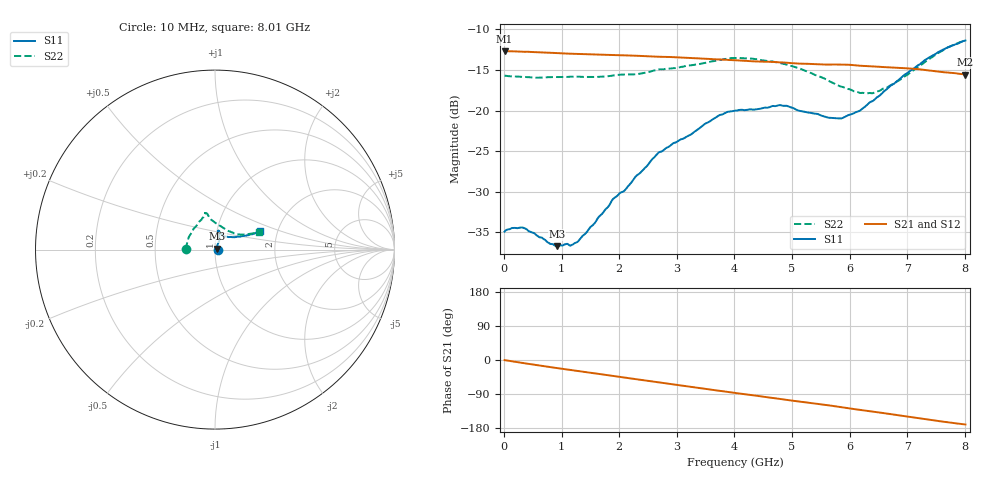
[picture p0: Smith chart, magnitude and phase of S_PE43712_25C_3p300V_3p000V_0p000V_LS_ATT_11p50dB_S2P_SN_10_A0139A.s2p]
! DEVICE ID: PE43712
! File Path: z:\PE43713\PE43713_CHAR_NOM_04292014\AMB\3p300\LS_ATT_11p50dB\PE43713_AMB_3p300V_3p000V_0p000V_LS_ATT_11p50dB_S2P_SN_10_A0139A.s2p
! Serial: 10
! Lot: A0139A
! Temp: 25C
! VDD: 3.300
! VSS: 0.000
! Control_Hi: 3.000
! Control_Lo: 0.000
! Attenuation Step: 11.50dB
! Port 1: RF1
! Port 2: RF2
! ThroughPath:1-2
! IDD: 0.0001469761
! ISS: -1.221e-007
#  Hz  S  RI  R  50
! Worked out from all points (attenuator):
!   801 points, 10 MHz to 8.01 GHz, reference 50 ohm
!   highest |S21| = -12.69 dB at 10 MHz (marker M1); lowest = -15.6 dB at 8.01 GHz (marker M2)
!   lowest |S11| = -36.7 dB at 920 MHz (marker M3), VSWR 1.03, Z = 51.4 + j0.509 ohm
!   |S11| at or under -10 dB: start of sweep to end of sweep
!   |S22| runs from -17.9 to -11.5 dB; largest |S21 - S12| = 0.00084
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1e7  0.018 0.000284  0.2321 -0.00123  0.2323 -0.00114  -0.164 0.00112
1.6e8  0.019 0.000579  0.2309 -0.0159  0.231 -0.0159  -0.1618 0.011
3.4e8  0.019 0.000202  0.2277 -0.0329  0.2277 -0.0323  -0.1597 0.0206
9.2e8  0.0138 0.00495  0.2104 -0.082  0.2105 -0.082  -0.1515 0.0537
1.18e9  0.0118 0.00909  0.1996 -0.101  0.1996 -0.1011  -0.1462 0.0689
1.35e9  0.0119 0.0118  0.192 -0.113  0.192 -0.113  -0.1415 0.0775
1.9e9  0.0139 0.0252  0.1628 -0.1475  0.1628 -0.1474  -0.1226 0.1099
2.1e9  0.0147 0.0289  0.1506 -0.1584  0.1506 -0.1583  -0.1163 0.1193
2.68e9  0.0232 0.0499  0.1113 -0.1833  0.1112 -0.1833  -0.0873 0.1565
3.72e9  0.0238 0.0897  0.0331 -0.2037  0.0329 -0.2036  -0.0577 0.1959
4.01e9  0.0222 0.0974  0.0113 -0.2038  0.0112 -0.2037  -0.0557 0.2033
4.79e9  0.0196 0.1062  -0.0438 -0.1931  -0.0439 -0.1933  -0.0399 0.1922
5.35e9  0.0299 0.0916  -0.0788 -0.1766  -0.0788 -0.1765  -0.0223 0.1677
5.64e9  0.0404 0.0808  -0.0952 -0.1669  -0.0952 -0.1669  -0.00156 0.1522
5.87e9  0.0505 0.0742  -0.1093 -0.1575  -0.1092 -0.1575  0.0184 0.1388
6.17e9  0.0703 0.0705  -0.1251 -0.1415  -0.1248 -0.1417  0.0496 0.1187
6.3e9  0.0827 0.0696  -0.1305 -0.1348  -0.1302 -0.1348  0.0647 0.1098
6.41e9  0.0914 0.0698  -0.135 -0.1289  -0.1347 -0.129  0.0766 0.1028
6.68e9  0.1201 0.0705  -0.1456 -0.1132  -0.1454 -0.1133  0.1086 0.0898
7.36e9  0.1926 0.0833  -0.163 -0.0684  -0.1629 -0.0685  0.1855 0.0871
7.72e9  0.2279 0.0933  -0.1651 -0.0454  -0.165 -0.0455  0.227 0.0951
8.01e9  0.2489 0.1049  -0.1642 -0.0287  -0.1641 -0.0289  0.2478 0.0995
